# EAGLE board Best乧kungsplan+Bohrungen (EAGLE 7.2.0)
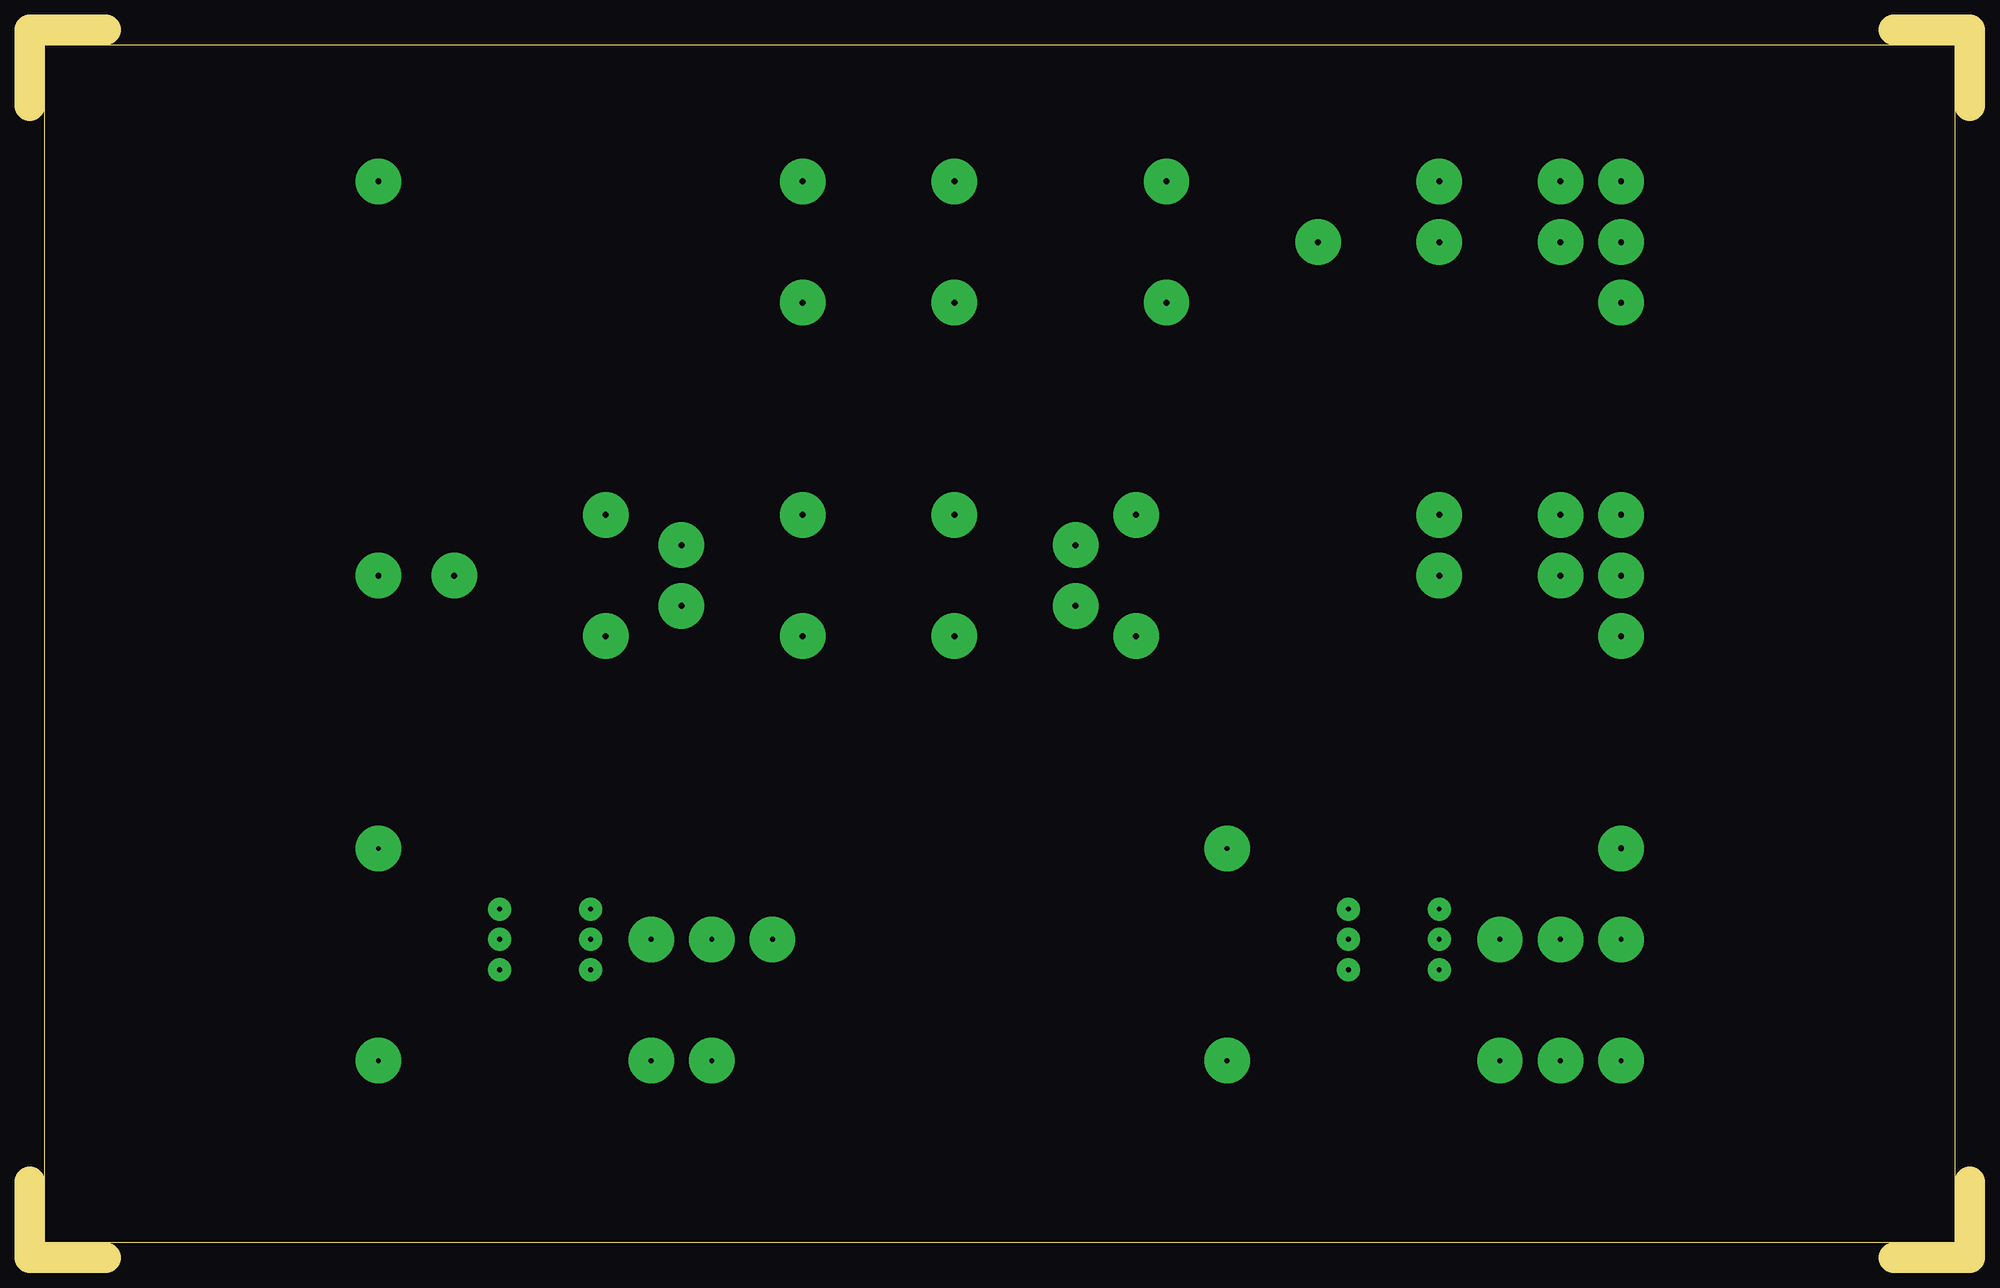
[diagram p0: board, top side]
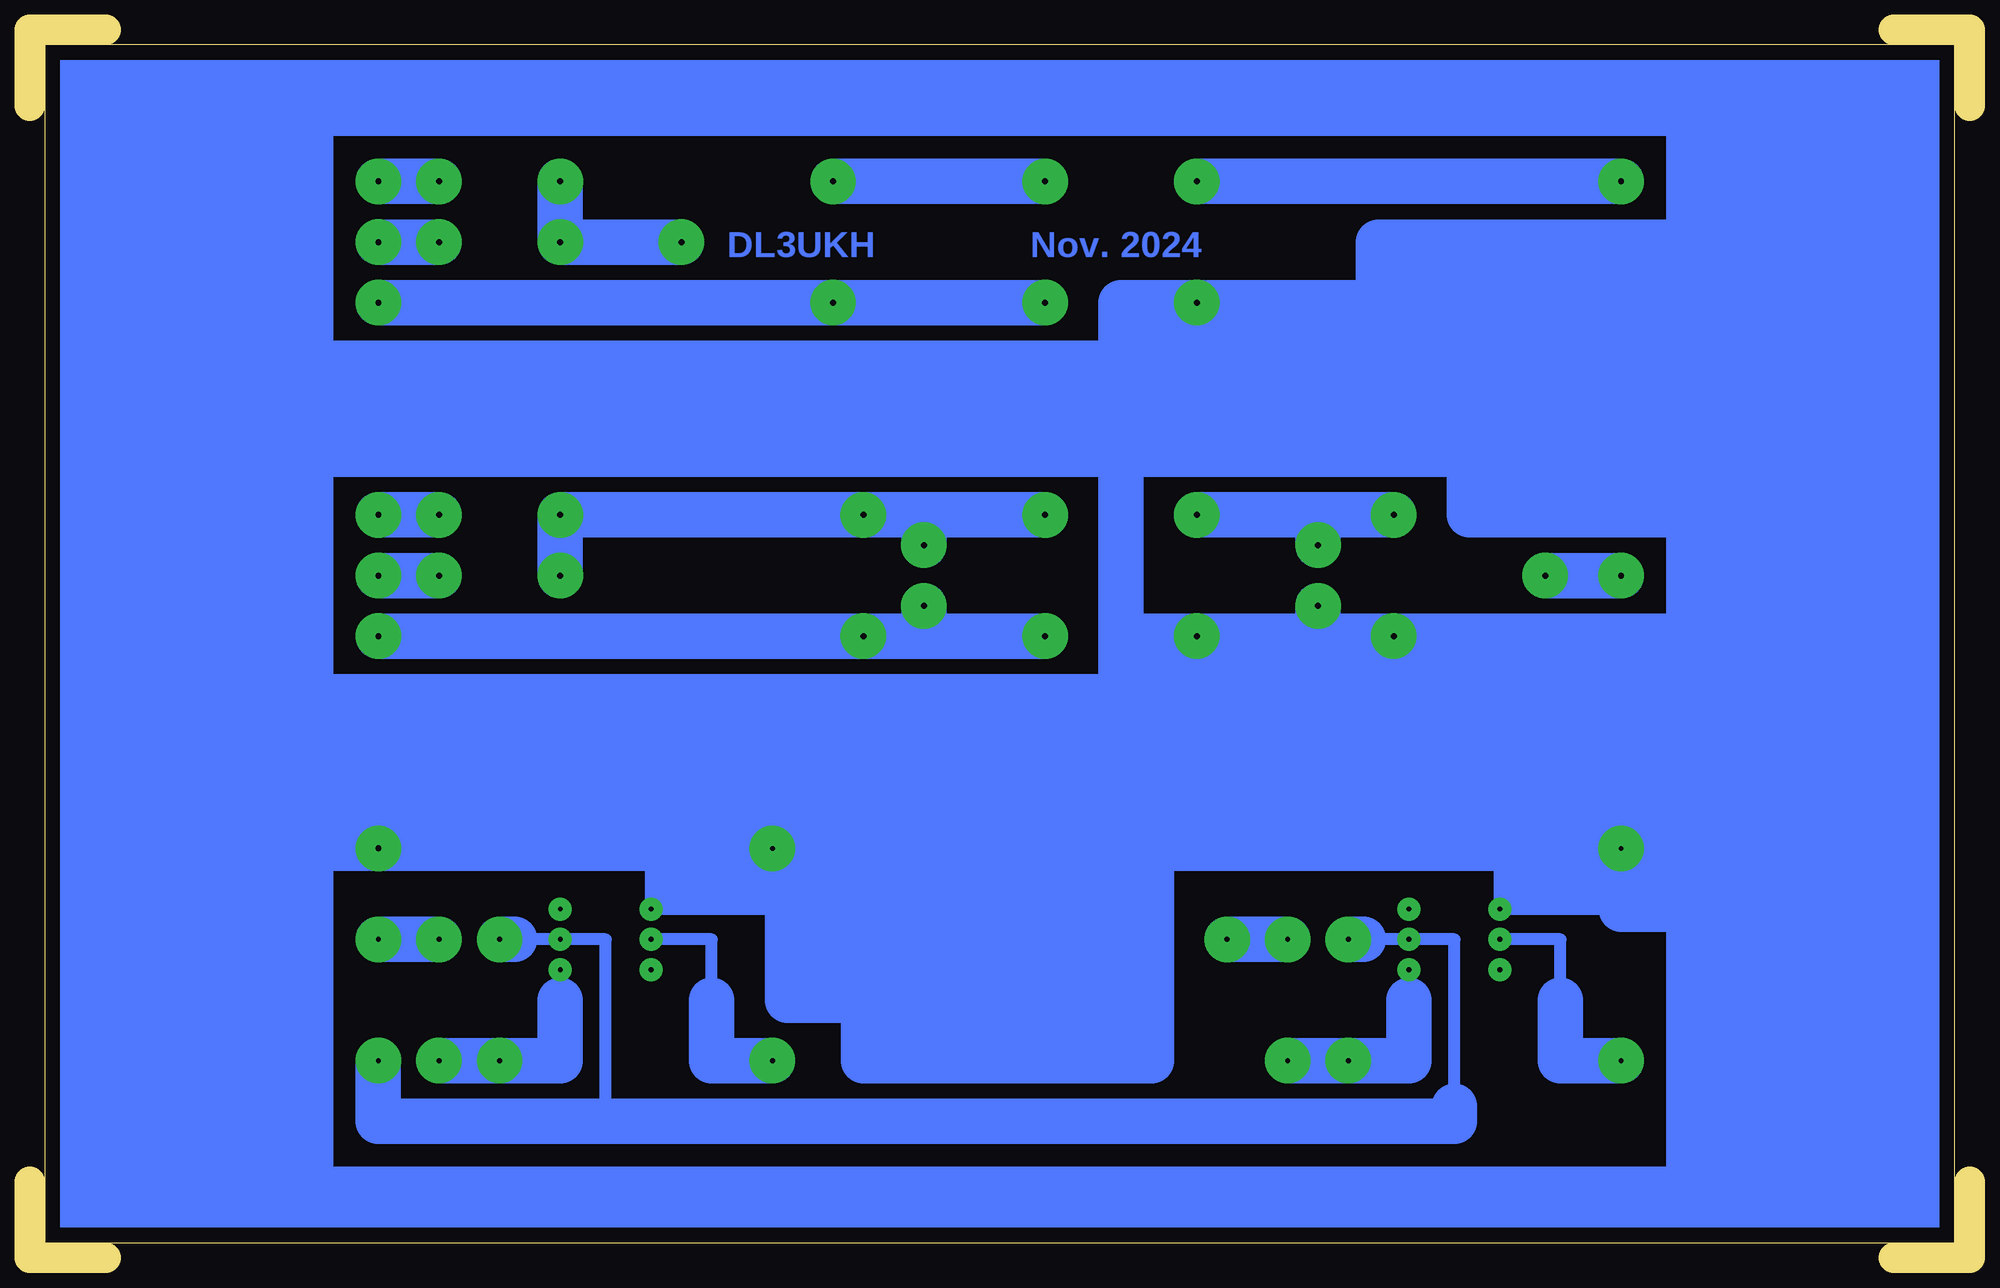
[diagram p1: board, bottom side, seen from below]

Size 162.56 x 102.87 mm. Coordinates in mm from the lower left corner, seen from the top.
Outline: 0,6.35 0,0 6.35,0
Outline: 0,96.52 0,102.87 6.35,102.87
Outline: 156.21,102.87 162.56,102.87 162.56,96.52
Outline: 162.56,6.35 162.56,0 156.21,0
Outline: 1.27,1.27 1.27,101.6 161.29,101.6 161.29,1.27 1.27,1.27
Copper layers 16: Bottom 0.035mm
Design rules "default": minimum track width 10mil, minimum drill 24mil, track to track 8mil, track to pad 8mil, pad to pad 8mil, via to via 8mil, smd to smd 8mil, copper to edge 40mil, drill to drill 8mil, minimum pad ring 10mil, minimum via ring 8mil, stop-mask expansion 4mil, vias tented up to drill 0mil, thermal gap 10mil

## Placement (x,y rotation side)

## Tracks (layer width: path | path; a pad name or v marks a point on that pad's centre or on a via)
S$1  (via drill 0.4 pad 1.93, 0.4 pad 3.81)
  Bottom 1.016: v39.37,26.67 34.29,26.67 34.29,21.59
  Bottom 3.81: v29.21,16.51 34.29,16.51 34.29,21.59
S$2  (via drill 0.4 pad 3.81)
  other vias: 128.27,26.67
S$3  (via drill 0.5 pad 3.81)
  Bottom 3.81: v77.47,90.17 87.63,90.17 v95.25,90.17
S$4  (via drill 0.4 pad 1.93)
  other vias: 39.37,24.13
S$5  (via drill 0.4 pad 1.93)
  other vias: 46.99,29.21
S$6  (via drill 0.4 pad 1.93, 0.4 pad 3.81)
  Bottom 1.016: 121.92,26.67 v118.11,26.67 114.3,26.67 114.3,11.43 | 50.8,26.67 v46.99,26.67 43.18,26.67 43.18,12.7 | 43.18,11.43 114.3,11.43 | 114.3,11.43 133.35,11.43
  Bottom 3.81: v133.35,16.51 133.35,11.43 43.18,11.43 43.18,12.7 | v52.07,26.67 50.8,26.67 | v123.19,26.67 121.92,26.67
S$7  (via drill 0.5 pad 3.81)
  Bottom 3.81: v48.26,62.23 54.61,62.23 | 54.61,62.23 v64.77,62.23 | v54.61,59.69 54.61,62.23
S$8  (via drill 0.4 pad 1.93, 0.4 pad 3.81)
  Bottom 1.016: v110.49,26.67 105.41,26.67 105.41,21.59
  Bottom 3.81: v100.33,16.51 105.41,16.51 105.41,21.59
S$9  (via drill 0.4 pad 1.93)
  other vias: 110.49,24.13
S$10  (via drill 0.4 pad 1.93)
  other vias: 118.11,29.21
S$11  (via drill 0.5 pad 3.81)
  Bottom 3.81: v77.47,80.01 87.63,80.01 v95.25,80.01 v133.35,80.01
S$12  (via drill 0.4 pad 1.93, 0.4 pad 3.81)
  Bottom 1.016: v118.11,24.13 118.11,21.59
  Bottom 3.81: v128.27,16.51 v123.19,16.51 118.11,16.51 118.11,21.59
S$13  (via drill 0.4 pad 1.93, 0.4 pad 3.81)
  Bottom 1.016: v46.99,24.13 46.99,21.59
  Bottom 3.81: v57.15,16.51 v52.07,16.51 46.99,16.51 46.99,21.59
S$14  (via drill 0.4 pad 3.81)
  Bottom 3.81: v57.15,26.67 v62.23,26.67 | 128.27,26.67 v133.35,26.67
S$15  (via drill 0.5 pad 3.81)
  Bottom 3.81: v107.95,85.09 v118.11,85.09 v118.11,90.17
S$16  (via drill 0.5 pad 3.81)
  Bottom 3.81: v29.21,90.17 54.61,90.17 v64.77,90.17
S$17  (via drill 0.4 pad 1.93, 0.4 pad 3.81, 0.5 pad 3.81)
  Bottom 1.016: 29.21,30.48 29.21,29.21 v39.37,29.21 39.37,34.29 | 105.41,29.21 v110.49,29.21 | 105.41,29.21 v100.33,34.29 100.33,29.21 | 105.41,34.29 105.41,29.21 | 100.33,29.21 v110.49,29.21 | v110.49,29.21 110.49,34.29 | 100.33,29.21 92.71,29.21
  Bottom 3.81: 41.91,67.31 140.97,67.31 140.97,74.93 71.12,74.93 | v133.35,34.29 110.49,34.29 105.41,34.29 v100.33,34.29 71.12,34.29 | 54.61,52.07 v48.26,52.07 | 54.61,52.07 v64.77,52.07 | 54.61,52.07 v54.61,54.61 | 71.12,34.29 71.12,52.07 | 71.12,52.07 71.12,74.93 | 71.12,74.93 71.12,80.01 v64.77,80.01 21.59,80.01 | 54.61,34.29 68.58,34.29 | 68.58,34.29 71.12,34.29 | 54.61,34.29 54.61,52.07 | v29.21,34.29 39.37,34.29 54.61,34.29 | 71.12,34.29 71.12,21.59 | 71.12,16.51 92.71,16.51 92.71,21.59 | 92.71,21.59 92.71,29.21 92.71,33.02 | v29.21,34.29 29.21,46.99 | 29.21,46.99 133.35,46.99 | 133.35,46.99 v133.35,34.29 | v29.21,34.29 29.21,30.48 | v48.26,52.07 48.26,45.72 | v64.77,52.07 64.77,45.72 | v64.77,52.07 71.12,52.07 | 92.71,21.59 99.06,21.59 99.06,30.48 | 92.71,21.59 71.12,21.59 | 71.12,21.59 71.12,16.51 | 71.12,16.51 68.58,16.51 68.58,34.29 | v48.26,52.07 29.21,52.07 | 29.21,52.07 29.21,46.99 | 133.35,46.99 140.97,46.99 | v133.35,34.29 140.97,34.29 | 29.21,29.21 20.32,29.21 20.32,52.07 29.21,52.07 | 41.91,67.31 41.91,62.23 22.86,62.23 22.86,67.31 41.91,67.31
S$18  (via drill 0.5 pad 3.81)
  Bottom 3.81: v128.27,85.09 v133.35,85.09
S$19  (via drill 0.5 pad 3.81)
  Bottom 3.81: v128.27,90.17 v133.35,90.17
S$20
  Bottom 3.81: 24.13,85.09 49.53,85.09 49.53,77.47
S$21  (via drill 0.5 pad 3.81)
  Bottom 3.81: v128.27,57.15 v133.35,57.15
S$22  (via drill 0.5 pad 3.81)
  Bottom 3.81: v128.27,62.23 v133.35,62.23
S$23  (via drill 0.5 pad 3.81)
  Bottom 3.81: v118.11,57.15 v118.11,62.23 v92.71,62.23 87.63,62.23 | v77.47,62.23 87.63,62.23 | 87.63,62.23 v87.63,59.69
S$24
  Bottom 3.81: 48.9,82.55 48.26,82.55
S$27  (via drill 0.5 pad 3.81)
  Bottom 3.81: v77.47,52.07 87.63,52.07 | 87.63,52.07 v92.71,52.07 v133.35,52.07 | v87.63,54.61 87.63,52.07
S$30  (via drill 0.5 pad 3.81)
  Bottom 3.81: v29.21,57.15 v35.56,57.15
(copper drawn outside any net)
  shapes: Bottom area x18

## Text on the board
Bottom: Nov. 2024 | DL3UKH
Pads: AUF BESTÜCKUNGS-SEITE GESEHEN
tOrigins: Optokoppler | 4N33 | ACHTUNG: | Leiterplatte: | Der Übertrager 1:5 muß | 1,5mm dick | 1N4148 | 1 | Cevausit | Die Aussparung | richtig herum einge- | Links oben ist | muß mit dem | lötet sein ! | immer PIN 1 | Bauelement | Alles mit 0,8mm vorbohren ! | und dem Bestück- | Man muß den Wider- | ungsplan | Aufbohren: | stand jeder Spule | überein stimmen. | Katode | Anode | Einstellregler 1,2mm | vorher messen ! | K | Übertrager 1,0mm | Siehe Beschreibung ! | Richtet sich nach der | Beschaltung des | nur Brücke | 680 | Buchse MAB 6 | Anschlußkabels | trcvr NF-Out | links | 10K | von hinten auf die Löt- | rechts | anschlüsse gesehen. | 680 | Buchse MAB 5S | Line In | Masse | von hinten auf die Löt- | anschlüsse gesehen. | nur Brücke | jetzt 1 : 1 | 680 | links | rechts | trcvr NF-In | 10K | 5 : 1 | 680 | 4,7n | 4,7n | 680 | Line Out | an Schalter | Masse | Richtet sich nach der | Beschaltung des | Gehäuse | Anschlußkabels | trcver-Masse | 4N33 | CW | 4N33 | Masse | RTS | an SUB-D-Stecker | Pin 7 | trcver-Masse | an Klinkenbuchse | DTR | an SUB-D-Stecker | Sub-D-Stecker | von hinten auf die Löt- | 1 | 1 | Pin 4 | 1N4148 | 1,5K | CW-trcvr | 1N4148 | 1,5K | anschlüsse gesehen. | an Klinkenbuchse | PTT-trcvr | K | K | Masse-PC | Pin5 | Pin1 | an SUB-D-Stecker | Pin 5 | Pin9 | Pin6 | Klinkenbuchse 3,5mm | Dies muß so | von hinten auf die Löt- | angeschlossen sein ! | anschlüsse gesehen. | Siehe Pin-Bezeichnung | auf der Leiterplatte !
